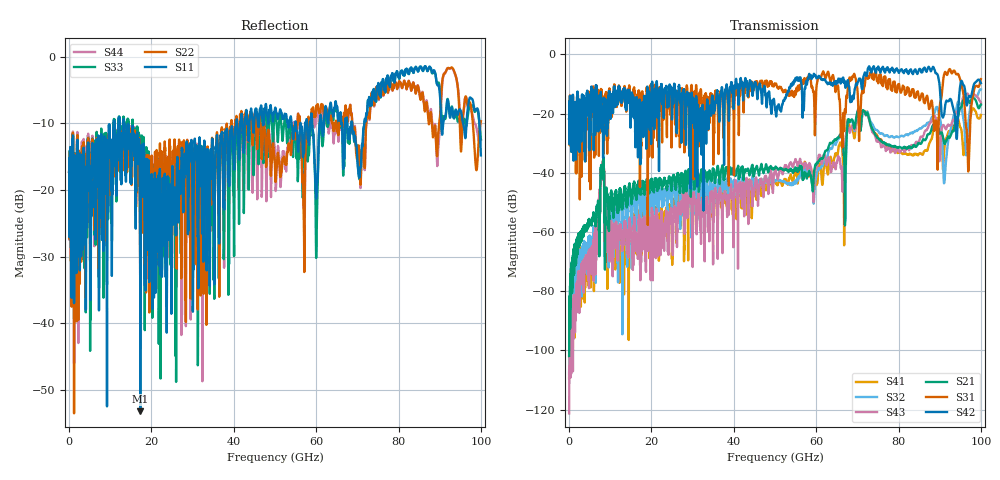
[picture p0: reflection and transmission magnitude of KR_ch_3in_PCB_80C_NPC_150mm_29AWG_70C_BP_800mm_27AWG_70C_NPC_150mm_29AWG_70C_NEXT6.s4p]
# GHz S RI R 45
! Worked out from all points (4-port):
!   4000 points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, 25 MHz to 100 GHz, reference 45 ohm
!   strongest paths, dB at 25 MHz, 25.02 GHz, 50.02 GHz, 75.03 GHz, 100 GHz:
!     S42: -21.8, -20.6, -18.8, -4.2, -9.7
!     S31: -21.8, -15.8, -10.0, -9.3, -8.4
!     S21: -101.9, -43.4, -38.3, -28.3, -17.0
!     S43: -121.3, -59.5, -39.5, -29.5, -16.4
!     S32: -107.9, -51.4, -42.9, -25.9, -11.9
!     S41: -109.5, -66.9, -43.0, -28.0, -20.5
!   lowest |S11| = -53.2 dB at 17.3 GHz (marker M1), VSWR 1.00, Z = 45.2 - j0.0837 ohm
!   |S11| at or under -10 dB: start of sweep to 10.89 GHz; 13.4 GHz to 40.64 GHz (27.24 GHz wide, 101 % of centre); 68.72 GHz to 71.7 GHz (2.978 GHz wide, 4.24 % of centre)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
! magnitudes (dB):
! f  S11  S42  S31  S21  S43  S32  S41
! 25 MHz  -17.3  -21.8  -21.8  -101.9  -121.3  -107.9  -109.5
! 8.05 GHz  -25.6  -23.2  -24.4  -40.7  -37.6  -39.4  -38.2
! 17.3 GHz  -53.2  -29.4  -22.4  -46.0  -70.0  -52.5  -58.5
! 72.05 GHz  -9.4  -7.1  -7.8  -20.3  -20.6  -20.4  -20.0
! 91.25 GHz  -9.0  -18.2  -6.1  -30.3  -24.8  -41.5  -30.2
! 96.85 GHz  -7.7  -15.3  -36.1  -15.2  -13.4  -24.4  -23.8
! 100 GHz  -14.8  -9.7  -8.4  -17.0  -16.4  -11.9  -20.5
